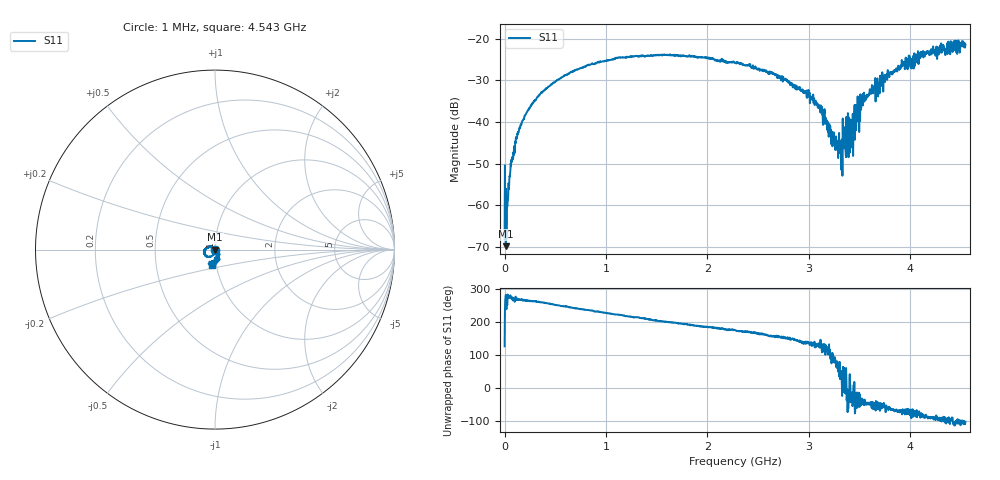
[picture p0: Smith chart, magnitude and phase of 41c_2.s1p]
# HZ S RI R 50
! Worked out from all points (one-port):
!   1515 points, 1 MHz to 4.543 GHz, reference 50 ohm
!   lowest |S11| = -69.9 dB at 13 MHz (marker M1), VSWR 1.00, Z = 50 - j0.0312 ohm
!   |S11| at or under -10 dB: start of sweep to end of sweep
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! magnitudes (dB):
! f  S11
! 1 MHz  -68.3
! 13 MHz  -69.9
! 58 MHz  -51.7
! 76 MHz  -48.4
! 127 MHz  -42.8
! 166 MHz  -40.6
! 340 MHz  -33.5
! 571 MHz  -29.2
! 1.138 GHz  -24.4
! 1.705 GHz  -24.0
! 2.272 GHz  -25.7
! 2.641 GHz  -28.5
! 2.842 GHz  -31.7
! 3.088 GHz  -36.5
! 3.163 GHz  -39.1
! 3.244 GHz  -44.6
! 3.31 GHz  -44.6
! 3.346 GHz  -46.3
! 3.355 GHz  -41.2
! 3.391 GHz  -48.5
! 3.409 GHz  -39.4
! 3.436 GHz  -48.2
! 3.457 GHz  -41.3
! 3.466 GHz  -41.9
! 3.541 GHz  -34.0
! 3.976 GHz  -26.6
! 4.219 GHz  -23.5
! 4.543 GHz  -21.4
